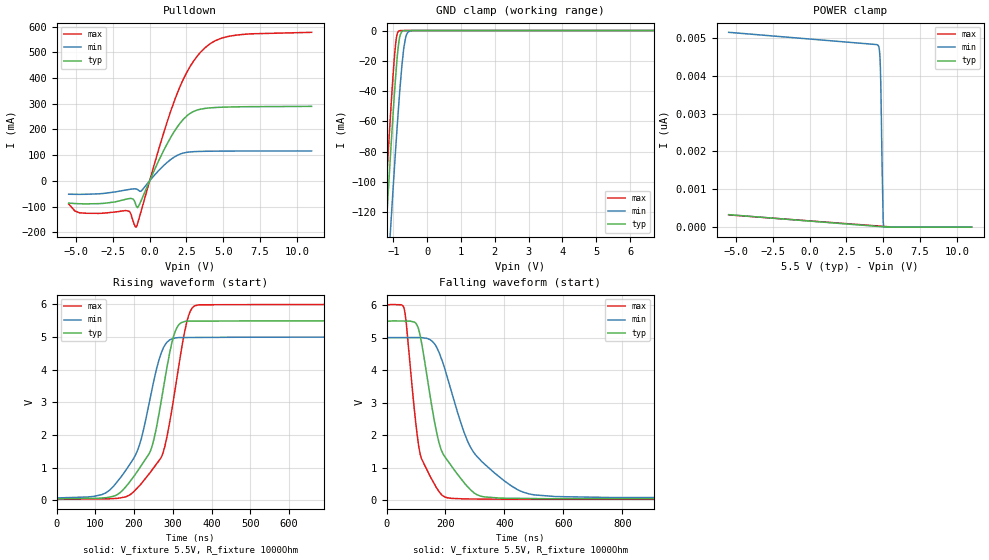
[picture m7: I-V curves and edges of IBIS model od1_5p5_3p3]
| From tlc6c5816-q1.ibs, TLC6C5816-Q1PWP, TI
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|   od1_5p5_3p3 Model
[Model]   od1_5p5_3p3
Model_type   Open_drain
Polarity   Inverting
Vmeas = 2.75
Vref = 5.5
Cref = 2pF
Rref = 1000
|   typ   min   max
C_comp   4.463pF   3.923pF   4.609pF
| Where Nom  PVT is Nominal Process, 5.5V, 27C
|   Fast PVT is Strong Process,  6.0V, -40C
|   Slow PVT is Weak Process,   5.0V, 150C
[Voltage Range]   5.5   5   6
|Junction Temperature
[Temperature Range]   27   150   -40
[Pullup Reference]   5.5   5   6
[Pulldown Reference]   0   -0   0
[Power Clamp Reference]   5.5   5   6
[GND Clamp Reference]   0   0   0
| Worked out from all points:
|   slope of the pulldown table from 0 to 0.825 V, typ, clamps not added: 8 ohm
|   GND clamp passes 1 mA (typ) near -0.76 V on its own axis
|   falling waveform, V_fixture 5.5V, R_fixture 1000Ohm: 20-80 % time 87.1ns typ, 141ns min, 48ns max; typ from 5.5 V to 0.041 V
|   rising waveform, V_fixture 5.5V, R_fixture 1000Ohm: 20-80 % time 67.7ns typ, 71.3ns min, 60.1ns max; typ from 0.041 V to 5.5 V
[Pulldown]
|   Voltage   I(typ)   I(min)   I(max)
-5.5V     -86.55mA   -52.18mA   -90mA
-4.758V   -89.21mA   -52.6mA    -124.4mA
-1.375V   -68.84mA   -33.33mA   -119mA
-913mV    -96.87mA   -31.84mA   -179.9mA
-583mV    -77.72mA   -39.99mA   -118.8mA
704mV     89mA       45.25mA    139.5mA
1.645V    189.4mA    91.44mA    305.5mA
2.552V    253.8mA    111mA      425mA
3.476V    278.9mA    114.5mA    501.4mA
4.4V      285mA      115.3mA    543.2mA
5.555V    287.3mA    115.7mA    564mA
11V       289.6mA    116.2mA    577.7mA
[GND Clamp]
|   Voltage   I(typ)   I(min)   I(max)
-5.5V     -1.93A     -1.907A    -1.997A
-1.375V   -193.6mA   -240.8mA   -169.5mA
-1.26V    -148.7mA   -197.1mA   -123.2mA
-1.194V   -123.4mA   -172.5mA   -97.38mA
-1.078V   -80.43mA   -130.2mA   -53.97mA
-995.5mV  -51.41mA   -100.8mA   -25.95mA
-929.5mV  -30.24mA   -78.14mA   -8.512mA
-830.5mV  -6.789mA   -46.41mA   -244.4uA
-682mV    -66.71uA   -10.45mA   -495.5nA
-599.5mV  -3.753uA   -2.242mA   -28.35nA
-451mV    -21.84nA   -64.6uA    -307pA
11V       0A         0A         0A
[POWER Clamp]
|   Voltage   I(typ)   I(min)   I(max)
-5.5V     329.9pA    5.145nA    324.3pA
4.631V    20.22pA    4.807nA    31.57pA
4.73V     17.33pA    4.699nA    28.77pA
4.763V    16.38pA    4.565nA    27.84pA
4.796V    15.43pA    4.299nA    26.91pA
4.829V    14.48pA    3.819nA    25.99pA
4.846V    14.01pA    3.484nA    25.52pA
4.912V    12.14pA    1.848nA    23.67pA
4.978V    10.29pA    530.8pA    21.83pA
4.994V    9.839pA    158.8pA    21.37pA
5.027V    8.939pA    0A         20.45pA
11V       0A         0A         0A
[Ramp]
R_load = 1000
|   typ   min   max
dV/dt_r   3.27522/6.74141e-08   2.9568/7.12304e-08   3.58243/6.00259e-08
dV/dt_f   3.27525/8.69729e-08   2.95685/1.4067e-07   3.58246/4.80064e-08
[Falling Waveform]
V_fixture = 5.5V
V_fixture_min = 5V
V_fixture_max = 6V
R_fixture = 1000Ohm
C_fixture = 0F
|   Time   V(typ)   V(min)   V(max)
0s        5.5V       5V         6V
59.48ns   5.508V     5V         5.893V
106.2ns   5.327V     5.001V     1.862V
118.4ns   4.861V     4.999V     1.284V
170.5ns   2.062V     4.696V     373.3mV
206ns     1.235V     3.784V     78.22mV
258.4ns   597.3mV    2.21V      44.65mV
296ns     234.4mV    1.469V     39.27mV
493.4ns   53.88mV    178.7mV    32.27mV
2.5us     41.25mV    71.92mV    29.23mV
[Rising Waveform]
V_fixture = 5.5V
V_fixture_min = 5V
V_fixture_max = 6V
R_fixture = 1000Ohm
C_fixture = 0F
|   Time   V(typ)   V(min)   V(max)
0s        41.25mV    71.92mV    29.23mV
117ns     70.51mV    174.2mV    42.86mV
170.5ns   306.6mV    781.9mV    86.96mV
213.8ns   980.7mV    1.691V     445.4mV
246.2ns   1.648V     3.397V     926.7mV
268.2ns   2.912V     4.449V     1.277V
309.1ns   5.257V     4.979V     3.641V
339.6ns   5.49V      4.988V     5.624V
364ns     5.491V     4.99V      5.985V
2.5us     5.5V       5V         6V
